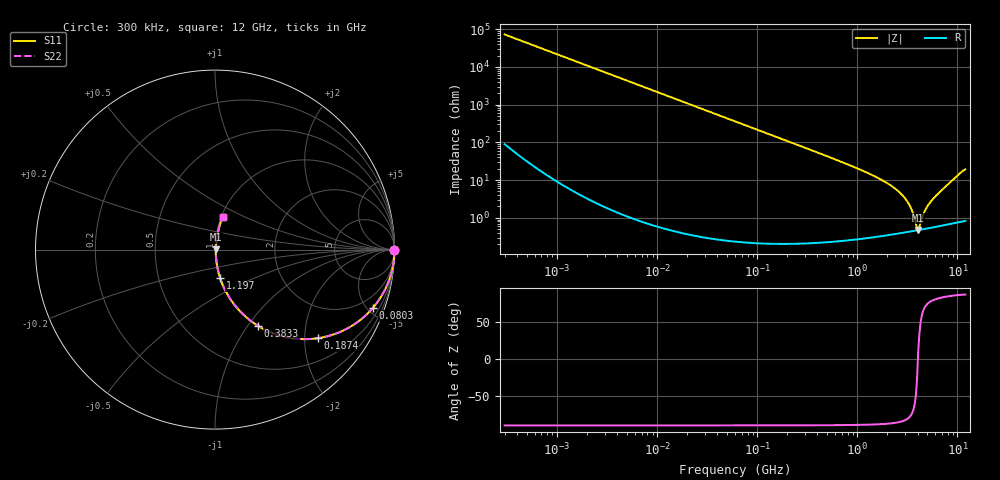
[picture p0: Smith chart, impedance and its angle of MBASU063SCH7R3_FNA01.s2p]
! MBASU063SCH7R3_FNA01  S-PARAMETER MODEL  ( General Type )
! Model Generated by TAIYO YUDEN Corporation (http://www.ty-top.com)
! Version 1.0
! TAIYO YUDEN Control No. 130801
! Copyright(c) 2013 TAIYO YUDEN CO.,LTD. All Rights Reserved.
! Product Description (link to TY-COMPAS)
! https://ds.yuden.co.jp/TYCOMPAS/or/detail?pn=MBASU063SCH7R3DFNA01&u=M
! Products Name : Multilayer Ceramic Capacitors
! Characteristics :
!  Capacitance : 7.3 pF , Rated Voltage : 50V , TCC : CH / C0H
!  Case Size : 0.6 x 0.3 / 0.024 x 0.012 [mm/inch] , Thickness : 0.3 / 0.012 [mm/inch]
!  (Conditions: Temperature = 25 degC , DC Bias Current/Voltage = 0A / 0V)
! External Node Assignments :
!  1  o---| |---o  2
! GND o---------o GND
! Frequency Range : 0.3MHz  -  12000MHz  [ 401 STEP ]
# MHz S RI R 50
! Freq[MHz].  S11 Real  S11 Imag  S21 Real  S21 Imag  S12 Real  S12 Imag  S22 Real  S22 Imag
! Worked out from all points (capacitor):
!   401 points, 300 kHz to 12 GHz, reference 50 ohm
!   read as one part in series: C = 7.32 pF near 316.3 kHz
!   lowest |Z| = 478 mohm at 4.05 GHz (marker M1)
!   series resonance near 4.024 GHz, so ESL is about 210 pH
!   S11 on the Smith chart (normalised r, x): 300 kHz: open; 80.3 MHz: 1.00, -5.41; 187.4 MHz: 1.00, -2.31; 383.3 MHz: 1.00, -1.12; 1.197 GHz: 1.01, -0.33; 12 GHz: 1.02, +0.38
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0.3  1 -0.00138  3.61e-06 0.00138  3.61e-06 0.00138  1 -0.00138
1.769972  0.9999 -0.00814  6.88e-05 0.00814  6.88e-05 0.00814  0.9999 -0.00814
10.44266  0.9977 -0.0479  0.00231 0.0479  0.00231 0.0479  0.9977 -0.0479
27.10171  0.9846 -0.1227  0.0154 0.1227  0.0154 0.1227  0.9846 -0.1227
60  0.9291 -0.2564  0.0709 0.2564  0.0709 0.2564  0.9291 -0.2564
80.29859  0.8797 -0.3249  0.1203 0.3249  0.1203 0.3249  0.8797 -0.3249
187.4445  0.5724 -0.4939  0.4276 0.4939  0.4276 0.4939  0.5724 -0.4939
353.9943  0.2715 -0.443  0.7285 0.443  0.7285 0.443  0.2715 -0.443
383.2761  0.241 -0.4258  0.759 0.4258  0.759 0.4258  0.241 -0.4258
634.0297  0.1023 -0.2995  0.8977 0.2995  0.8977 0.2995  0.1023 -0.2995
1197.383  0.0293 -0.1603  0.9707 0.1603  0.9707 0.1603  0.0293 -0.1603
2088.533  0.00921 -0.0753  0.9908 0.0753  0.9908 0.0753  0.00921 -0.0753
2650.866  0.00601 -0.0462  0.994 0.0462  0.994 0.0462  0.00601 -0.0462
3107.553  0.00495 -0.0283  0.9951 0.0283  0.9951 0.0283  0.00495 -0.0283
3454.93  0.00463 -0.0167  0.9954 0.0167  0.9954 0.0167  0.00463 -0.0167
3841.137  0.0046 -0.00532  0.9954 0.00532  0.9954 0.00532  0.0046 -0.00532
4050.141  0.00469 0.000795  0.9953 -0.000795  0.9953 -0.000795  0.00469 0.000795
4270.516  0.00484 0.0054  0.9952 -0.0054  0.9952 -0.0054  0.00484 0.0054
4875.354  0.00541 0.0168  0.9946 -0.0168  0.9946 -0.0168  0.00541 0.0168
5565.855  0.00629 0.0285  0.9937 -0.0285  0.9937 -0.0285  0.00629 0.0285
9454.42  0.0201 0.1124  0.9799 -0.1124  0.9799 -0.1124  0.0201 0.1124
12000  0.0429 0.1822  0.9571 -0.1822  0.9571 -0.1822  0.0429 0.1822
